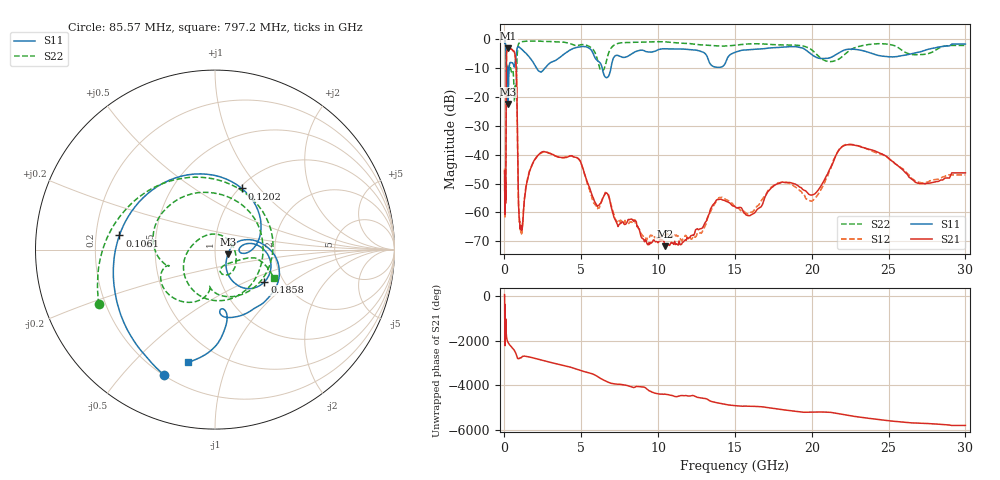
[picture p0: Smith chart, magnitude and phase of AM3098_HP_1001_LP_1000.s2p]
! Date/Time: Thu, Feb 28, 2019 8:41 AM
! Network Analyzer: Agilent Technologies E8364B Rev: A.07.50.67
! Sweep from 0.010 to 30.000 GHz, 1601 Points, Sweep Type: LOG
! Power Supply: 5.022 V, 0.002 A
# Hz S DB R 50
!freq MagS11 AngS11 MagS21 AngS21 MagS12 AngS12 MagS22 AngS22
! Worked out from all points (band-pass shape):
!   1601 points, 10 MHz to 30 GHz, reference 50 ohm
!   highest |S21| = -2.99 dB at 256 MHz (marker M1); lowest = -71.7 dB at 10.44 GHz (marker M2)
!   |S21| within 3 dB of the highest: 130.2 MHz to 706.2 MHz (576 MHz wide, 138 % of centre)
!   lowest |S11| = -22.3 dB at 239.9 MHz (marker M3), VSWR 1.17, Z = 57.7 - j2.95 ohm
!   |S11| at or under -10 dB: 191.2 MHz to 304.5 MHz (113.3 MHz wide, 45.7 % of centre); 2.092 GHz to 2.621 GHz (528.7 MHz wide, 22.4 % of centre); 6.366 GHz to 6.928 GHz (561.8 MHz wide, 8.45 % of centre)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
!   |S22| runs from -21.3 to -0.5 dB; largest |S21 - S12| = 0.0084
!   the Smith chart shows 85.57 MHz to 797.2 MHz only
!   S11 on the Smith chart (normalised r, x): 85.57 MHz: 0.20, -0.65; 106.1 MHz: 0.30, +0.07; 120.2 MHz: 1.03, +0.81; 185.8 MHz: 1.60, -0.65; 797.2 MHz: 0.34, -0.73
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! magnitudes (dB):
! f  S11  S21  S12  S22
! 10 MHz  -0.3  -45.6  -44.8  -0.6
! 38.04 MHz  -0.5  -59.3  -61.4  -0.9
! 49.1 MHz  -0.7  -52.5  -49.4  -1.2
! 85.57 MHz  -2.5  -55.0  -53.2  -2.9
! 106.1 MHz  -5.4  -28.5  -28.6  -6.9
! 120.2 MHz  -8.6  -10.8  -10.8  -10.0
! 144.7 MHz  -17.1  -4.3  -4.3  -13.2
! 185.8 MHz  -9.7  -3.5  -3.5  -8.9
! 239.9 MHz  -22.3  -3.0  -3.0  -11.3
! 256 MHz  -18.3  -3.0  -2.9  -10.9
! 550.5 MHz  -8.3  -3.9  -3.8  -11.0
! 655.8 MHz  -9.3  -4.5  -4.5  -21.3
! 797.2 MHz  -3.8  -15.6  -15.5  -8.8
! 917.1 MHz  -2.5  -57.3  -57.5  -1.5
! 1.066 GHz  -3.1  -64.7  -67.2  -0.9
! 2.084 GHz  -9.9  -40.8  -40.8  -0.6
! 4.71 GHz  -2.8  -41.0  -41.1  -2.1
! 7.926 GHz  -6.1  -63.9  -63.4  -1.0
! 10.44 GHz  -3.2  -71.7  -68.0  -0.8
! 20 GHz  -5.2  -54.0  -56.1  -3.6
! 22.56 GHz  -3.3  -36.5  -36.4  -3.5
! 30 GHz  -1.6  -46.3  -47.0  -2.0
